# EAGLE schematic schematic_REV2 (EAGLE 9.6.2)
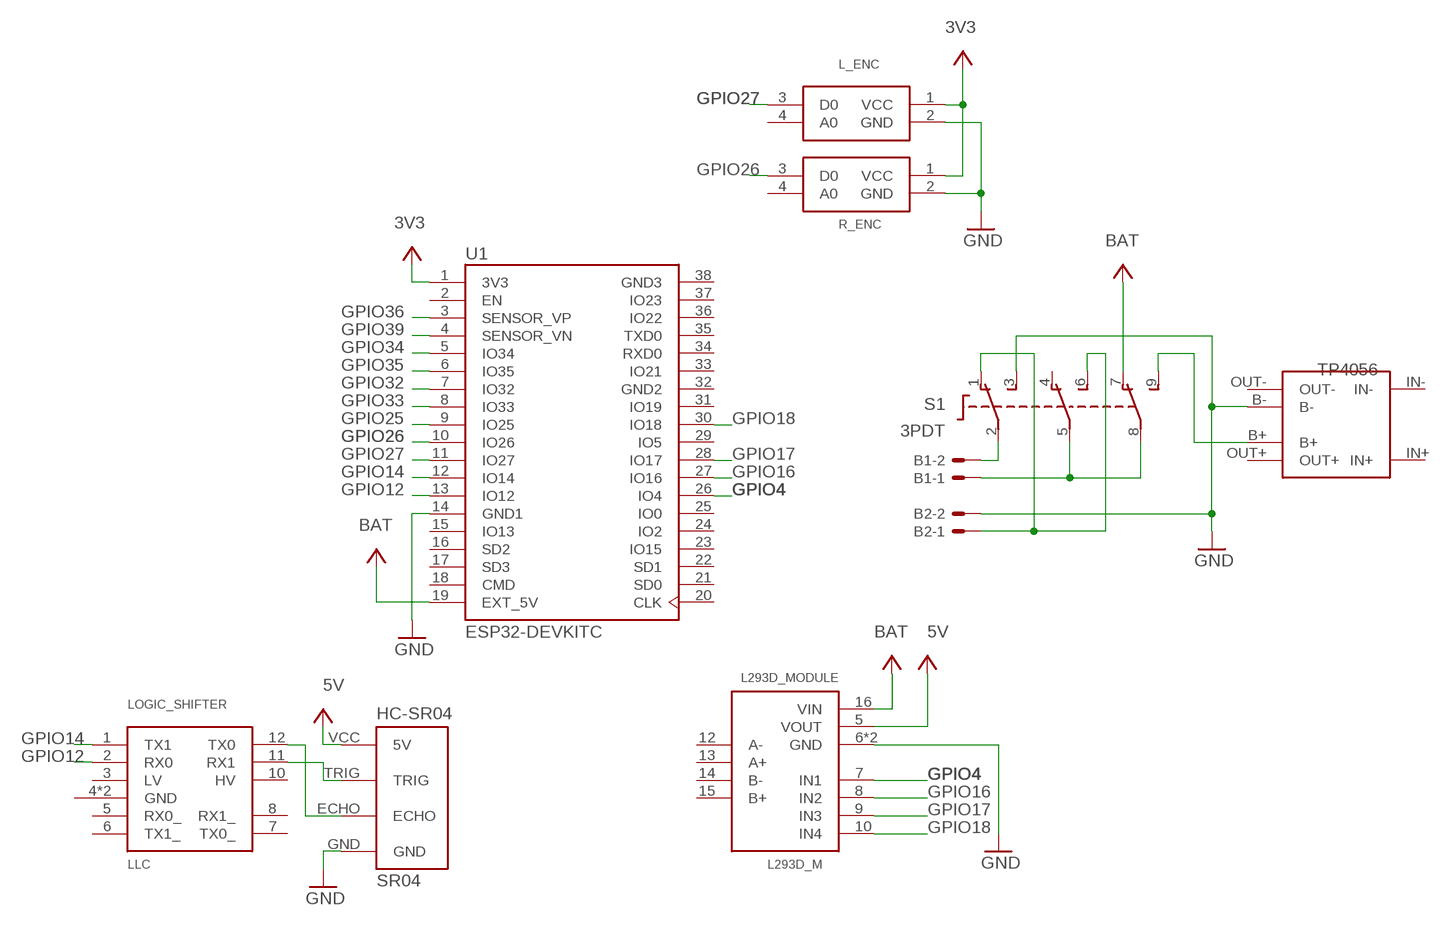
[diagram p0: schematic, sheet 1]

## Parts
B1  22-23-2021  [22-23-2021]
B2  22-23-2021  [22-23-2021]
BAT_CHARGER  TP4056-MODULE  [TP4056-LITHIUM-PROTECTED-MODULE]
L293D_MODULE  L293D_M  [L293D_M]
L_ENC  ENCODER  [ENCODER]
LOGIC_SHIFTER  LLC  [LLC]
R_ENC  ENCODER  [ENCODER]
S1  3PDT  [3PDT]
SR04  HC-SR04  [HC-SR04_FOOTPRINT]
U1  ESP32-DEVKITC  [MODULE_ESP32-DEVKITC]

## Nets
GND: B2.2 BAT_CHARGER.B- L293D_MODULE.6(GND) L293D_MODULE.11(GND) S1.3(S1) SR04.GND U1.14(GND1)
GPIO4 [Signals]: L293D_MODULE.7(IN1) U1.26(IO4)
GPIO12: LOGIC_SHIFTER.2(RX0) U1.13(IO12)
GPIO14: LOGIC_SHIFTER.1(TX1) U1.12(IO14)
GPIO16 [Signals]: L293D_MODULE.8(IN2) U1.27(IO16)
GPIO17 [Signals]: L293D_MODULE.9(IN3) U1.28(IO17)
GPIO18 [Signals]: L293D_MODULE.10(IN4) U1.30(IO18)
GPIO25: U1.9(IO25)
GPIO26: R_ENC.3(D0) U1.10(IO26)
GPIO27: L_ENC.3(D0) U1.11(IO27)
GPIO32: U1.7(IO32)
GPIO33: U1.8(IO33)
GPIO34: U1.5(IO34)
GPIO35: U1.6(IO35)
GPIO36: U1.3(SENSOR_VP)
GPIO39: U1.4(SENSOR_VN)
N$1: B1.2 S1.2(P1)
N$2: B2.1 S1.1(O1) S1.6(S2)
N$3: LOGIC_SHIFTER.12(TX0) SR04.ECHO
N$4: BAT_CHARGER.B+ S1.9(S3)
N$5: B1.1 S1.5(P2) S1.8(P3)
N$6: L_ENC.2(GND) R_ENC.2(GND) ; supply symbol labelled GND
N$7: LOGIC_SHIFTER.11(RX1) SR04.TRIG
VCC: L293D_MODULE.5(VOUT) L293D_MODULE.16(VIN) L_ENC.1(VCC) R_ENC.1(VCC) S1.7(O3) SR04.VCC(5V) U1.1(3V3) U1.19(EXT_5V)
Unconnected: L293D_MODULE.12(A-) L293D_MODULE.13(A+) L293D_MODULE.14(B-) L293D_MODULE.15(B+) L_ENC.4(A0) LOGIC_SHIFTER.3(LV) LOGIC_SHIFTER.4(GND) LOGIC_SHIFTER.5(RX0_) LOGIC_SHIFTER.6(TX1_) LOGIC_SHIFTER.7(TX0_) LOGIC_SHIFTER.8(RX1_) LOGIC_SHIFTER.9(GND) LOGIC_SHIFTER.10(HV) R_ENC.4(A0) S1.4(O2) U1.2(EN) U1.15(IO13) U1.16(SD2) U1.17(SD3) U1.18(CMD) U1.20(CLK) U1.21(SD0) U1.22(SD1) U1.23(IO15) U1.24(IO2) U1.25(IO0) U1.29(IO5) U1.31(IO19) U1.33(IO21) U1.34(RXD0) U1.35(TXD0) U1.36(IO22) U1.37(IO23)

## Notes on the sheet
- TP4056

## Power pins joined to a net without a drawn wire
GND2: U1.32(GND2)
GND3: U1.38(GND3)
IN+: BAT_CHARGER.IN+
IN-: BAT_CHARGER.IN-
OUT+: BAT_CHARGER.OUT+
OUT-: BAT_CHARGER.OUT-

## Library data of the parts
B1 B2 = con-molex:22-23-2021: .100" (2.54mm) Center Header - 2 Pin; MF: MOLEX; MPN: 22-23-2021; OC_FARNELL: 1462926; OC_NEWARK: 25C3832
BAT_CHARGER = UserLib:TP4056-MODULE
L293D_MODULE = edurobotParts:L293D_M
L_ENC R_ENC = edurobotParts:ENCODER
LOGIC_SHIFTER = edurobotParts:LLC
S1 = switch:3PDT: 3PDT 9 pin footswitch SF17020F-0302-21R-L Source: 3PDT.jpg
SR04 = Ultrasonic Sensor HC-SR04:HC-SR04: Ultrasonic Sensor HC-SR04
U1 = ESP32-DEVKITC:ESP32-DEVKITC: ESP32-DEVKITC Check availability; AVAILABILITY: In Stock; DESCRIPTION: ESP32-WROOM32 series Transceiver; 802.11 b/g/n (Wi-Fi, WiFi, WLAN), Bluetooth® Smart 4.x Low Energy (BLE) Evaluation Board; MF: Olimex LTD; MP: ESP32-DEVKITC; PACKAGE: None; PRICE: None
